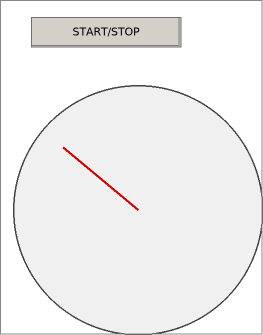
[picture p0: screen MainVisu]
VISUALIZATION MainVisu  // 263x335
    Button (31,17 150x30), "START/STOP"
        toggle MAIN.bRun
    Meter360 (13,85 250x250), value: MAIN.fGaugeValue, style: Meter-Meter360-Gray, scale format: %.1f, scale 0..100
END_VISUALIZATION
